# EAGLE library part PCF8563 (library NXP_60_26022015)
Real time clock/calendar The PCF8563 is a CMOS Real-Time Clock (RTC) and calendar optimized for low power consumption. A programmable clock output, interrupt output, and voltage-low detector are also provided. All addresses and data are transferred serially via a two-line bidirectional I2C-bus. Maximum bus speed is 400 kbit/s. The register address is incremented automatically after each written or read data byte. AAL Eindhoven MK
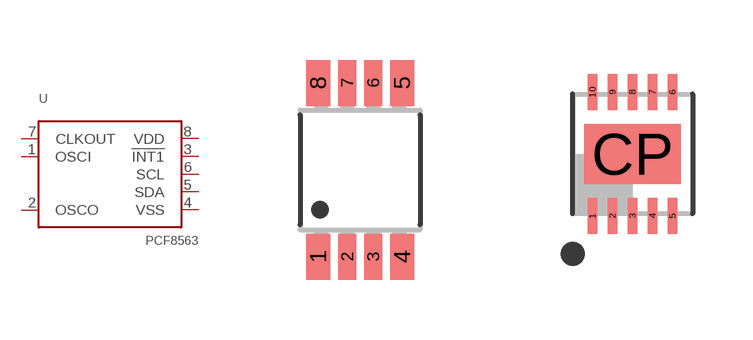
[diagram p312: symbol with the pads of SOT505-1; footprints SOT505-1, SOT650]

Designator prefix U

## PCF8563TS  [SOT505-1]
1  OSCI  pas
2  OSCO  pas
3  !INT1!  out
4  VSS  pwr
5  SDA
6  SCL  in
7  CLKOUT  pwr
8  VDD  pwr

## PCF8563BS  [SOT650]
1  OSCI  pas
2  OSCO  pas
4  !INT1!  out
5  VSS  pwr
6  SDA
7  SCL  in
8  CLKOUT  pwr
9  VDD  pwr

## PCF8563P  [SOT97-1]
Pads as for SOT505-1

## PCF8563T  [SOT96-1]
Pads as for SOT505-1

## Footprint SOT505-1 (pad centres in mm)
SOT505-1 TSSOP8: plastic thin shrink small outline package; 8 leads; body width 3 mm JEDEC: -- IEC: --
smd 0.6 x 1.15: 1 -1.05,-2.175; 4 1.05,-2.175; 5 1.05,2.175; 8 -1.05,2.175
smd 0.45 x 1.15: 2 -0.325,-2.175; 3 0.325,-2.175; 6 0.325,2.175; 7 -0.325,2.175

## Footprint SOT650 (pad centres in mm)
SOT650 HVSON10: plastic thermal enhanced very thin small outline package; no leads; 10 terminals; body 3 x 3 x 0.85 mm JEDEC: MO-229 IEC: -- JEITA:--
smd 0.24 x 0.9: 1 -1,-1.55; 2 -0.5,-1.55; 3 0,-1.55; 4 0.5,-1.55; 5 1,-1.55; 6 1,1.55; 7 0.5,1.55; 8 0,1.55; 9 -0.5,1.55; 10 -1,1.55
smd 2.4 x 1.5: CP 0,0

## Footprint SOT97-1 (pad centres in mm)
Dual In Line Package
drill 0.813 long: 1 -3.81,-3.81; 2 -1.27,-3.81; 3 1.27,-3.81; 4 3.81,-3.81; 5 3.81,3.81; 6 1.27,3.81; 7 -1.27,3.81; 8 -3.81,3.81

## Footprint SOT96-1 (pad centres in mm)
SOT96-1 SO8: plastic small outline package; 8 leads; body width 3.9 mm JEDEC: MS-012 IEC: 076E03
smd 0.6 x 1.3: 1 -1.905,-2.65; 2 -0.635,-2.65; 3 0.635,-2.65; 4 1.905,-2.65; 5 1.905,2.65; 6 0.635,2.65; 7 -0.635,2.65; 8 -1.905,2.65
